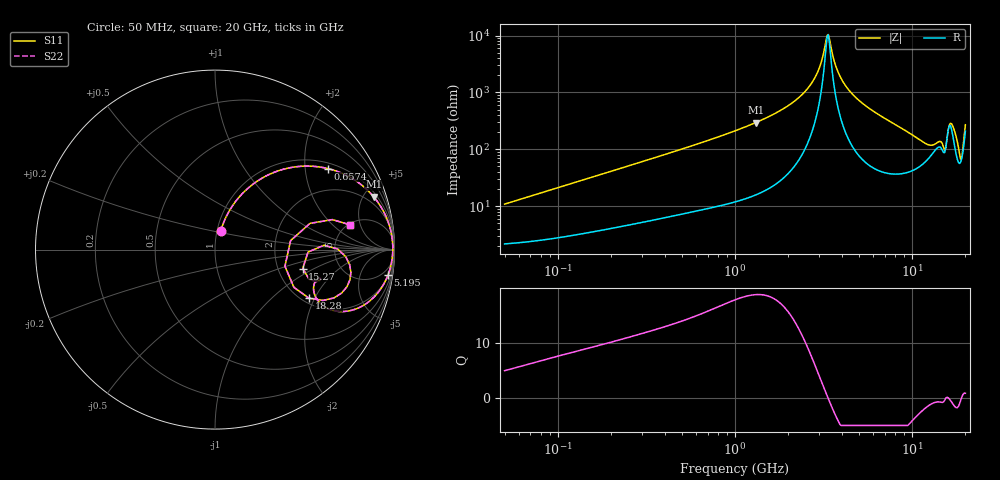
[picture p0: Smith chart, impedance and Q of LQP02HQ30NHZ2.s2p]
!Murata Part Number: LQP02HQ30NHZ2
!These Parameters are Measured in Series Mode Connection
!  o--[Z]--o
!Port1  Port2
!  o-------o
!Freq. Start=50[MHz] Stop=20[GHz], 401[Steps]
# Hz S RI R 50
!Freq.(Hz) S11(Real) S11(Imag) S21(Real) S21(Imag) S12(Real) S12(Imag) S22(Real) S22(Imag)
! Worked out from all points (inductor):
!   401 points, 50 MHz to 20 GHz, reference 50 ohm
!   read as one part in series: L = 33.8 nH near 51.52 MHz
!   highest Q = 18.7 at 1.309 GHz (marker M1), where L = 35.8 nH
!   self-resonance near 3.314 GHz
!   S11 on the Smith chart (normalised r, x): 50 MHz: 1.04, +0.21; 657.4 MHz: 1.17, +2.66; 5.195 GHz: 2, -13; 15.27 GHz: 2.75, -0.77; 18.28 GHz: 2.17, -1.80; 20 GHz: 5.17, +3.44
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5e7  0.0318 0.101  0.9682 -0.101  0.9682 -0.101  0.0318 0.101
1.364002e8  0.0995 0.2471  0.9005 -0.2471  0.9005 -0.2471  0.0995 0.2471
3.721004e8  0.3707 0.4448  0.6293 -0.4448  0.6293 -0.4448  0.3707 0.4448
6.574395e8  0.6313 0.4509  0.3687 -0.4509  0.3687 -0.4509  0.6313 0.4509
1e9  0.8032 0.3704  0.1968 -0.3704  0.1968 -0.3704  0.8032 0.3704
1.309461e9  0.8843 0.2942  0.1157 -0.2942  0.1157 -0.2942  0.8843 0.2942
2.083303e9  0.9666 0.149  0.0334 -0.149  0.0334 -0.149  0.9666 0.149
2.728004e9  0.9867 0.0643  0.0133 -0.0643  0.0133 -0.0643  0.9867 0.0643
2.98453e9  0.9896 0.0362  0.0104 -0.0362  0.0104 -0.0362  0.9896 0.0362
3.265178e9  0.9907 0.00796  0.00933 -0.00796  0.00933 -0.00796  0.9907 0.00796
3.364474e9  0.9906 -0.00149  0.00938 0.00149  0.00938 0.00149  0.9906 -0.00149
3.680849e9  0.9892 -0.03  0.0108 0.03  0.0108 0.03  0.9892 -0.03
3.967106e9  0.9865 -0.054  0.0135 0.054  0.0135 0.054  0.9865 -0.054
5.194772e9  0.9633 -0.1432  0.0367 0.1432  0.0367 0.1432  0.9633 -0.1432
7.442007e9  0.8811 -0.2691  0.1189 0.2691  0.1189 0.2691  0.8811 -0.2691
1.082228e10  0.6558 -0.3383  0.3442 0.3383  0.3442 0.3383  0.6558 -0.3383
1.527346e10  0.4886 -0.1057  0.5114 0.1057  0.5114 0.1057  0.4886 -0.1057
1.646126e10  0.7499 -0.0829  0.2501 0.0829  0.2501 0.0829  0.7499 -0.0829
1.721783e10  0.7356 -0.2062  0.2644 0.2062  0.2644 0.2062  0.7356 -0.2062
1.828096e10  0.5226 -0.2703  0.4774 0.2703  0.4774 0.2703  0.5226 -0.2703
1.912117e10  0.4212 0.0501  0.5788 -0.0501  0.5788 -0.0501  0.4212 0.0501
2e10  0.7527 0.1379  0.2473 -0.1379  0.2473 -0.1379  0.7527 0.1379
